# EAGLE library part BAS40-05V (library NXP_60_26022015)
General-purpose Schottky diodes General-purpose Schottky diodes in small Surface-Mounted Device (SMD) plastic packages. AAL Eindhoven MK
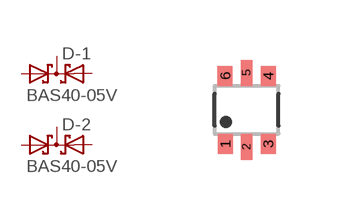
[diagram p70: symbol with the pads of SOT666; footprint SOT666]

Designator prefix D; gates -1=DIODE_SDD_AKKA -2=DIODE_SDD_AKKA

## BAS40-05V  [SOT666]
1  -1:A1  pas
2  -1:A2  pas
3  -2:K1K2  pas
4  -2:A1  pas
5  -2:A2  pas
6  -1:K1K2  pas

## Footprint SOT666 (pad centres in mm)
SOT 666 Reflow soldering foorprint Source: Philips - BAS70_1PS7XSB70_SER_8.pdf
smd 0.375 x 0.5: 1 -0.537,-0.85; 3 0.538,-0.85; 4 0.538,0.85; 6 -0.538,0.85
smd 0.3 x 0.65: 2 0,-0.925; 5 0,0.925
